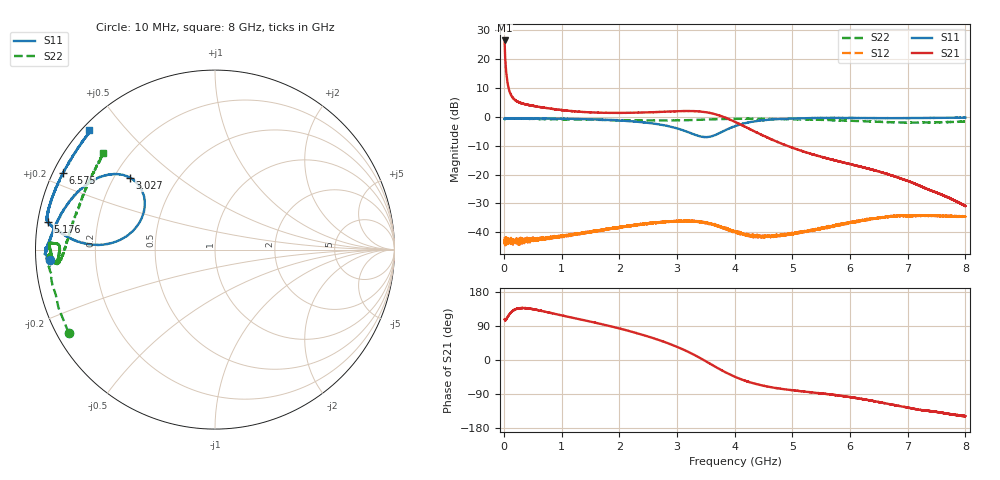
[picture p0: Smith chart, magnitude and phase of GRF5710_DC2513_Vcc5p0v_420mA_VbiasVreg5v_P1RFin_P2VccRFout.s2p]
!Keysight Technologies,N5244B,MY57181157,A.18.40.03
!Date: Thursday, September 18, 2025 15:54:06
!Correction: S11(C  2-Port  )
!S21(C  2-Port  )
!S12(C  2-Port  )
!S22(C  2-Port  )
!S2P File: Measurements: S11, S21, S12, S22:
# Hz S  RI  R 50
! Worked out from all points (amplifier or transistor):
!   7991 points, 10 MHz to 8 GHz, reference 50 ohm
!   highest |S21| = 26.4 dB at 10 MHz (marker M1)
!   |S21| within 3 dB of that: start of sweep to 14.22 MHz
!   unconditionally stable (mu >= 1): 115.1 MHz to 117.2 MHz; 126.4 MHz to 143.9 MHz; 144.3 MHz to end of sweep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
!   at 1.341 GHz: K = 1.89, MAG = 15.5 dB, |S12| = -40.2 dB
!   at 4.005 GHz: K = 5.38, MAG = 8.7 dB, |S12| = -39.7 dB
!   at 8 GHz: K = 17.54, MAG = -13.6 dB, |S12| = -34.5 dB
!   S11 on the Smith chart (normalised r, x): 10 MHz: 0.04, -0.03; 3.027 GHz: 0.26, +0.34; 5.176 GHz: 0.03, +0.08; 6.575 GHz: 0.03, +0.24; 8 GHz: 0.02, +0.40
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1e7  -0.9175 -0.0602  -6.361 19.95  0.00659 0.00117  -0.8157 -0.4627
5e7  -0.9366 -0.0105  -1.556 4.277  0.00729 0.000189  -0.9267 -0.0945
5.5e7  -0.9381 -0.0027  -1.504 3.869  0.00699 0.00052  -0.9201 -0.0906
6.1e7  -0.9413 -0.0144  -1.548 3.536  0.00796 0.00036  -0.9261 -0.0846
7.4e7  -0.9385 -0.00539  -1.482 2.944  0.00772 0.000389  -0.9261 -0.0737
9.1e7  -0.9416 -0.00319  -1.435 2.446  0.00756 -0.000472  -0.9255 -0.0592
1.13e8  -0.9396 0.00249  -1.375 2.04  0.00674 0.000874  -0.922 -0.0472
1.42e8  -0.9406 0.00124  -1.375 1.728  0.00688 6.31e-05  -0.9304 -0.0381
2.21e8  -0.9423 0.00567  -1.308 1.315  0.00772 0.000624  -0.9217 -0.0295
3.52e8  -0.9399 0.00553  -1.22 1.134  0.0077 0.00047  -0.9248 -0.0346
1.342e9  -0.9089 0.0861  -0.3441 1.167  0.00918 0.00223  -0.8869 -0.0702
2.674e9  -0.6161 0.4127  0.7233 0.9703  0.014 -0.00504  -0.8656 0.00385
3.027e9  -0.473 0.3997  1.047 0.6789  0.012 -0.01  -0.8673 0.0257
3.484e9  -0.4047 0.1859  1.205 -0.0448  0.00172 -0.0149  -0.8911 0.0347
3.752e9  -0.5291 0.0539  0.939 -0.4452  -0.00576 -0.0107  -0.9132 0.0363
4.005e9  -0.6889 0.0283  0.5827 -0.5708  -0.00914 -0.00497  -0.9192 0.0356
4.465e9  -0.8587 0.0954  0.1919 -0.4477  -0.00783 0.00359  -0.9205 0.00531
5.176e9  -0.9312 0.1544  0.0316 -0.2516  -0.00424 0.00903  -0.8965 -0.0662
5.337e9  -0.9382 0.1635  0.0182 -0.2254  -0.0042 0.0102  -0.8893 -0.0742
6.575e9  -0.8489 0.426  -0.0422 -0.0989  0.00376 0.018  -0.8066 0.1076
6.669e9  -0.8304 0.4549  -0.0442 -0.0904  0.00487 0.0181  -0.7972 0.1427
8e9  -0.7029 0.6666  -0.0243 -0.0152  0.0124 0.0143  -0.6213 0.5407
